FUNCTION_BLOCK FB_SimpleNciSequence
VAR_INPUT
	bExecute			: BOOL;						(*触发位*)
	bConfirmHsk			: BOOL	:= FALSE;			(*确认H握手代码*)
	sPrgName			: STRING(255) ;				(*G代码所在地址*)
END_VAR
VAR_OUTPUT
	bBusy				: BOOL;						(*功能块在被执行*)
	bError				: BOOL;						(*出现报错*)
	bDone				: BOOL;						(*功能块被执行完毕*)
END_VAR
VAR_IN_OUT
	stX					: AXIS_REF;					(*通道的X轴*)
	stY					: AXIS_REF;					(*通道的Y轴*)
	stZ					: AXIS_REF;					(*通道的Z轴*)
	st_Q1				: AXIS_REF;					(*通道的辅助Q1轴*)
	st_Q2				: AXIS_REF;					(*通道的辅助Q2轴*)
	st_Q3				: AXIS_REF;					(*通道的辅助Q3轴*) 
	stItpToPlc			: NCTOPLC_NCICHANNEL_REF;	(*NCI通道反馈给PLC的*)
	stPlcToItp			: PLCTONC_NCICHANNEL_REF;	(*PLC发送给NCI通道的*)
END_VAR
VAR
	nState				: UDINT	:= 0;				
	nErrorState			: UDINT;
	
	fbBuildGroup		: CfgBuildExt3DGroup;		(*创建通道，并将轴添加进通道*)
	fbLoadGCode			: ItpLoadProgEx;			(*装载G代码*)
	fbStartGCode		: ItpStartStopEx;			(*开始执行G代码*)
	fbClearGroup		: CfgReconfigGroup;			(*清除NCI通道中的周，释放轴*)
	fbConfirmHsk		: ItpConfirmHsk;			(*确认H握手代码*)
	
	nInterpreterState	: UDINT	:= 0;
	
	
END_VAR

CASE nState OF
0:
	IF bExecute THEN			(*功能块的触发位一旦触发后，执行以下：*)
		bBusy	:= TRUE;		(*FB为执行状态*)
		bDone	:= FALSE;		(*对执行完毕功能快的引脚复位*)
		bError	:= FALSE;		(*报错引脚复位*)
		nErrorState	:= nState;	(*nstate为0，认为无报错*)
		nState	:= 10;			(*进入10步*)
	END_IF	
	
10:
	// 该步用来将NC轴添加进NCI通道中
	fbBuildGroup(
		bExecute:=TRUE, 
		nGroupId:=ItpGetGroupId(sNciToPlc:=stItpToPlc) , 
		nXAxisId:=stX.NcToPlc.AxisId, 
		nYAxisId:=stY.NcToPlc.AxisId, 
		nZAxisId:=stZ.NcToPlc.AxisId, 
		nQ1AxisId:=st_Q1.NcToPlc.AxisId, 
		nQ2AxisId:=st_Q2.NcToPlc.AxisId, 
		nQ3AxisId:=st_Q3.NcToPlc.AxisId, 
		nQ4AxisId:= 0, 
		nQ5AxisId:= 0, 
		tTimeOut:= , 
		bBusy=> , 
		bErr=> , 
		nErrId=> );
	IF NOT fbBuildGroup.bBusy THEN
		IF NOT fbBuildGroup.bErr THEN
			nState	:= 20;(*如果将NC轴添加进NCI通道中成功后，进入20步*)
		ELSE
			(* add error handling *)
			nErrorState	:= nState;(*如果出现报错，首先FB出现报错，然后将错误状态定位在10步，并且进入9999步*)
			bBusy	:= FALSE;
			bError	:= TRUE;
			nState	:= 9999;
		END_IF
		fbBuildGroup(bExecute:=FALSE); (*对fbBuildGroup的触发位复位*)
	END_IF
	
20:
	(*将G代码装在进通道，sPrgName有两种用法，第一种写出路径+G代码程序的文件名，第二种直接写G代码程序的文件名,但需要放置在安装盘中TwinCAT\MC\NCI的文件夹*)
	// load g-code file 
	// pls. ensure that first.nc is available in TwinCAT\MC\NCI-folder 
	fbLoadGCode(
		sNciToPlc:=stItpToPlc, 
		bExecute:=TRUE, 
		sPrg:= sPrgName, 
		nLength:= INT_TO_UDINT(LEN(sPrgName)), 
		tTimeOut:= , 
		bBusy=> , 
		bErr=> , 
		nErrId=> );
	IF NOT fbLoadGCode.bBusy THEN
		IF NOT fbLoadGCode.bErr THEN
			nState	:= 30;(*如果装载G代码成功后，进入20步*)
		ELSE
			(* add error handling *)
			nErrorState	:= nState;(*如果出现报错，首先FB出现报错，然后将错误状态定位在20步，并且进入9999步*)
			bBusy	:= FALSE;
			bError	:= TRUE;
			nState	:= 9999;				
		END_IF
		fbLoadGCode(sNciToPlc:=stItpToPlc, bExecute:=FALSE); (*对fbLoadGCode的触发位复位*)
	END_IF
	
30:
	(*检查通道状态，如果处于ready，那么说明装载G代码成功*)
	// we have to check the status of the interpreter. It has to be in ready state, in case of loading the program successfully.
	nInterpreterState	:= ItpGetStateInterpreter(sNciToPlc:=stItpToPlc);(*获取通道当前状态*)
	IF nInterpreterState = Tc2_NCI.NCI_INTERPRETER_READY THEN(*判断通道是否为ready状态*)
		nState	:= 40;
	ELSE
		(* add error handling *)
		nErrorState	:= nState;(*如果通道没有到ready状态，将错误状态定位在30步，并且进入9999步*)
		bBusy	:= FALSE;
		bError	:= TRUE;
		nState	:= 9999;				
	END_IF
	
40:
	(*开始执行G代码*)
	// start g-code file
	fbStartGCode(
		bStart:=TRUE, 
		bStop:=FALSE, 
		tTimeOut:= , 
		sNciToPlc:= stItpToPlc, 
		bBusy=> , 
		bErr=> , 
		nErrId=> );
	IF NOT fbStartGCode.bBusy THEN
		IF NOT fbStartGCode.bErr THEN(*如果开始执行G代码了，进入50步*)
			nState	:= 50;
		ELSE	
			(* add error handling *)
			nErrorState	:= nState;(*如果未能成功执行，将错误状态定位在40步，并且进入9999步*)
			bBusy	:= FALSE;
			bError	:= TRUE;
			nState	:= 9999;				
		END_IF
		fbStartGCode( bStart:=FALSE, sNciToPlc:= stItpToPlc ); (*对fbStartGCode的触发位复位*)
	END_IF
	
50:
	(*检查状态，确认G代码是否执行完毕*)
	// check state, again - we are at least not in ready state for several ticks
	// this is to ensure that we don't indicate program has finished, before we have started 
	nInterpreterState	:= ItpGetStateInterpreter(sNciToPlc:=stItpToPlc);
	IF nInterpreterState <> Tc2_NCI.NCI_INTERPRETER_READY THEN(*判断通道是否为ready状态*)
		// nci is running
		nState	:= 60;(*不为ready的状态，进入60步*)
	END_IF

60:
	(*获取通道的当前状态*)
	nInterpreterState	:= ItpGetStateInterpreter(sNciToPlc:=stItpToPlc);
	IF	nInterpreterState = Tc2_NCI.NCI_INTERPRETER_READY THEN(*判断是否回到ready状态，回到说明G代码已经执行完毕,进入70步*)
		// program has finished
		nState	:= 70;
	ELSIF nInterpreterState = Tc2_NCI.NCI_INTERPRETER_ABORTED THEN(*如果通道状态变成aborted的话，说明通道此时出现报错，具体需要通过通道报错的ID进行排查原因*)
		// a run-time error occured - this could be a lag error or something else... 
		// add error handling
		;
	END_IF	
70:
	(*G代码执行完毕，释放NC轴，解散NCI通道*)
	// program has finished 
	// now clear interpolation group 
	fbClearGroup(
		bExecute:=TRUE, 
		nGroupId:=ItpGetGroupId(sNciToPlc:=stItpToPlc) , 
		tTimeOut:= , 
		bBusy=> , 
		bErr=> , 
		nErrId=> );
	IF NOT fbClearGroup.bBusy THEN
		IF NOT fbClearGroup.bErr THEN(*如果释放完毕，进入80步*)
			nState	:= 80;
		ELSE
			(* add error handling *)
			nErrorState	:= nState;(*如果未能成功执行，将错误状态定位在70步，并且进入9999步*)
			bBusy	:= FALSE;
			bError	:= TRUE;
			nState	:= 9999;				
		END_IF
		fbClearGroup(bExecute:=FALSE); (*对fbClearGroup的触发位复位*)
	END_IF
80:
	(*以上已经完成该功能块的目标，对输出位DONE置为TRUE，说明已完成G代码的执行*)
	bDone	:= TRUE;
	bBusy	:= FALSE;
	IF NOT bExecute THEN(*若此功能块的触发位没有复位，那么nState回到0步*)
		nState	:= 0;
	END_IF
9999:
	// error state 
	IF NOT bExecute THEN(*若此功能块的触发位没有复位,那么回到初始0步，重新执行*)
		nState	:= 0;
		bError	:= FALSE;
	END_IF
END_CASE

// handling of m-functions is done outside statemachine
// all m-functions are directly confiremd. In a real application we have of course to consider the m-function numbers to turn on/off certain functions in the machine.
(*原程序部分对H握手型直接做了复位，将此部分屏蔽，保留确认功能块
IF ItpIsHskMFunc(stItpToPlc) AND NOT fbConfirmHsk.bBusy THEN
	bConfirmHsk	:= TRUE;
ELSE	
	bConfirmHsk	:= FALSE;
END_IF	
*)

(*一旦G代码中出现M握手型，用于进行确认M握手指令*)
fbConfirmHsk(
	bExecute:=bConfirmHsk , 
	sNciToPlc:=stItpToPlc , 
	sPlcToNci:=stPlcToItp , 
	bBusy=> , 
	bErr=> , 
	nErrId=> );

END_FUNCTION_BLOCK
